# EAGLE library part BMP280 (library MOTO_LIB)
BAROMETER BMP280
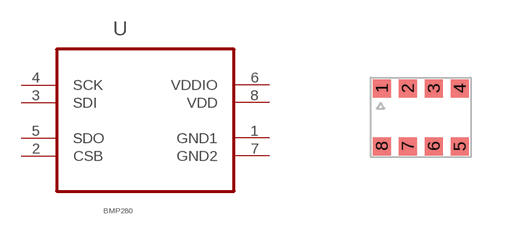
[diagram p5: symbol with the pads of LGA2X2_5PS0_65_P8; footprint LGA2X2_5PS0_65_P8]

Designator prefix U

## BMP280 (MPN: BMP280; SUPPLIER: BOSCH)  [LGA2X2_5PS0_65_P8]
1  GND1  pwr
2  CSB  in
3  SDI
4  SCK  in
5  SDO
6  VDDIO  pwr
7  GND2  pwr
8  VDD  pwr

## Footprint LGA2X2_5PS0_65_P8 (pad centres in mm)
smd 0.45 x 0.45: 1 -0.975,0.725; 2 -0.325,0.725; 3 0.325,0.725; 4 0.975,0.725; 5 0.975,-0.725; 6 0.325,-0.725; 7 -0.325,-0.725; 8 -0.975,-0.725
